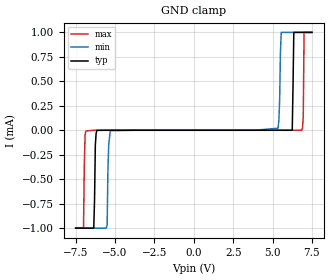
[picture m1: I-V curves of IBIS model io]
|Texas Instruments Incorporated
|ESD224 Low Clamping 4-Channel ESD Protection Device for HDMI Interface
[IBIS Ver]   4.1
[File name]   esd224.ibs
[Date]   01/29/2018
[File Rev]   1.0
[Source]
| Texas Instruments Incorporated.
| Analog-eLab Design Center, HPA
| 12500 TI Blvd
| Dallas, TX -75243
[Notes]
| Rev 1.0: 01/29/2018
| - Initial version of the model
| - Warnings regarding combined Non-monotonicity of various models
|   have been reviewed and considered minor and can be ignored.
[Disclaimer]
| This model is designed as an aid for customers of Texas Instruments.
| TI and its licensors and suppliers make no warranties, either expressed
| or implied, with respect to this  model, including the warranties of
| merchantability or fitness for a particular purpose. The model is
| provided solely on an "as is" basis. The entire risk as to its quality
| and performance is with the customer.
| This model is subject to change without notice. Texas Instruments
| Incorporated is not responsible for updating this model.
[Copyright]
(C) Copyright 2018 Texas Instruments Incorporated.All rights reserved.
|  Component ESD224DQA 10-pin USON - DQA package
|  Part # ESD224DQA
[Component]   ESD224DQA
[Manufacturer]  TI
[Package]   |10 USON - DQA package
|   typ   min   max
R_pkg   0.01   0.008   0.012
L_pkg   0.1nH   0.08nH   0.12nH
C_pkg   0.1pF   0.08pF   0.12pF
[Pin]  signal_name model_name   R_pin   L_pin   C_pin
1   IO1_C   io   NA   NA   NA
2   IO2_C   io   NA   NA   NA
3   GND   gnd   NA   NA   NA
4   IO3_C   io   NA   NA   NA
5   IO4_C   io   NA   NA   NA
6   IO4_S   io   NA   NA   NA
7   IO3_S   io   NA   NA   NA
8   GND   gnd   NA   NA   NA
9   IO2_S   io   NA   NA   NA
10   IO1_S   io   NA   NA   NA
| Models and submodels in the file (1): io (Terminator)
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|   io Model
[Model]   io
Model_type   Terminator
|   typ   min   max
C_comp   0.4pF   0.4pF   0.4pF
| Where Nom  PVT is Nominal Process, 7.2V, 25C
|   Fast PVT is Strong Process,  7.5V, -40C
|   Slow PVT is Weak Process,   7.0V, 125C
[Voltage Range]   7.2   7.0   7.5
|Junction Temperature
[Temperature Range]   25   125   -40
[Power Clamp Reference]   7.2   7.0   7.5
[GND Clamp Reference]   0   0   0
[GND Clamp]
|   Voltage   I(typ)   I(min)   I(max)
-7.5V     -1mA       -999.9uA   -1mA
-7V       -1mA       -999.9uA   -1mA
-6.85V    -1mA       -999.9uA   -7.77uA
-6.15V    -862nA     -999.9uA   -1.01nA
-5.3V     -1.1nA     -4.46uA    -186pA
5.35V     1.67nA     20.6uA     472pA
5.55V     2.42nA     1mA        583pA
6.25V     21.8nA     1mA        1.7nA
6.35V     1mA        1mA        2.06nA
6.85V     1mA        1mA        30.6nA
7V        1mA        1mA        1mA
7.5V      1mA        1mA        1mA
